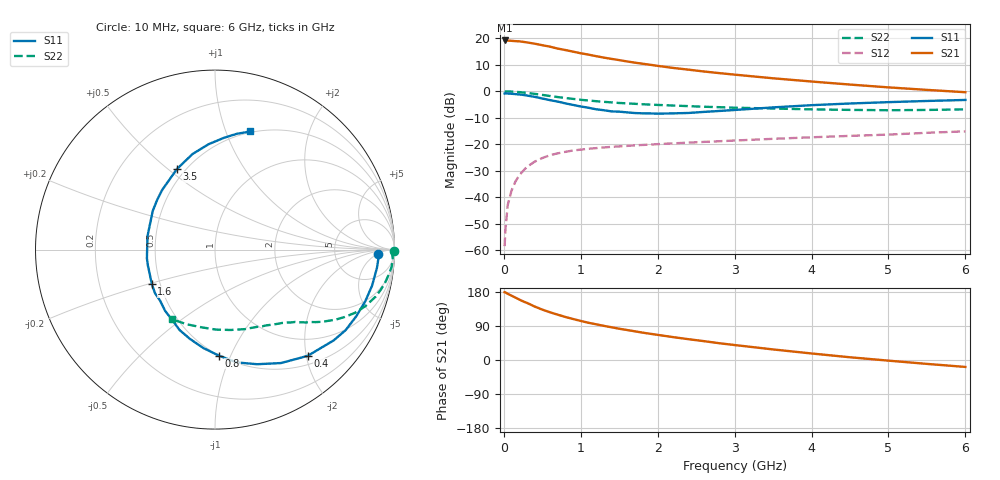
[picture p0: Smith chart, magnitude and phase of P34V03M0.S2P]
! SIEMENS Small Signal Semiconductors
! BFP181
! Si NPN RF Bipolar Junction Transistor in SOT143
! VCE = 4 V  IC = 3 mA
! Common Emitter S-Parameters:  March  1996
# GHz  S  MA  R  50
!  f  S11  S21  S12  S22
! GHz  MAG  ANG  MAG  ANG  MAG  ANG  MAG  ANG
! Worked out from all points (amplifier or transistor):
!   36 points, 10 MHz to 6 GHz, reference 50 ohm
!   highest |S21| = 19.2 dB at 10 MHz (marker M1)
!   |S21| within 3 dB of that: start of sweep to 690.9 MHz
!   unconditionally stable (mu >= 1): 2.142 GHz to end of sweep
!   at 250 MHz: K = 0.15, MSG = 24.3 dB, |S12| = -30.0 dB
!   at 1.4 GHz: K = 0.75, MSG = 16.6 dB, |S12| = -21.0 dB
!   at 6 GHz: K = 1.10, MAG = 5.5 dB, |S12| = -15.1 dB
!   lowest NFmin = 1.40 dB at 450 MHz
!   S11 on the Smith chart (normalised r, x): 10 MHz: 19, -5; 400 MHz: 0.66, -2.03; 800 MHz: 0.50, -0.91; 1.6 GHz: 0.45, -0.21; 3.5 GHz: 0.45, +0.54; 6 GHz: 0.49, +1.22
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0.01  0.9066 -1.5  9.092 178.9  0.0012 94.9  0.9953 -0.5
0.02  0.9122 -2.8  9.069 178.3  0.0024 86.2  0.987 -1.1
0.05  0.9081 -6.4  9.032 174.8  0.0071 89.4  0.9915 -2.9
0.1  0.898 -12.9  8.948 169.8  0.0134 82.4  0.9885 -5.7
0.2  0.87 -25.3  8.757 159.6  0.026 75.5  0.9653 -11.1
0.25  0.8554 -31.6  8.555 154.7  0.0315 72.0  0.9491 -13.8
0.4  0.7856 -48.9  7.902 141.2  0.047 63.0  0.8952 -20.6
0.5  0.7313 -59.8  7.398 133.0  0.0551 57.1  0.8558 -24.3
0.6  0.6804 -69.8  6.943 125.9  0.0623 53.2  0.815 -27.4
0.7  0.6399 -79.2  6.388 119.6  0.0676 49.5  0.779 -30.0
0.8  0.5913 -87.8  5.996 113.6  0.0721 45.9  0.7466 -32.1
1  0.517 -105.6  5.211 103.1  0.0794 41.0  0.6923 -35.7
1.1  0.4895 -113.8  4.92 98.2  0.0824 39.0  0.6694 -37.1
1.3  0.4398 -129.3  4.318 90.1  0.0873 35.7  0.6328 -39.8
1.6  0.4007 -151.5  3.658 79.2  0.0933 32.9  0.5924 -43.1
1.8  0.3843 -166.6  3.316 72.3  0.0972 31.8  0.5703 -45.4
2.2  0.3834 168.9  2.758 60.4  0.1043 29.1  0.5385 -50.3
2.8  0.4254 139.1  2.203 44.3  0.1143 26.6  0.5017 -58.5
3.5  0.4969 115.2  1.759 27.9  0.1269 23.8  0.4732 -69.5
4.5  0.5886 93.4  1.339 7.2  0.1442 19.3  0.4457 -89.4
5.5  0.6567 79.3  1.063 -10.3  0.1649 15.6  0.4449 -110.8
6  0.6867 73.4  0.96 -18.3  0.1756 12.7  0.4564 -121.9
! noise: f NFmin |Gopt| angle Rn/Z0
0.45  1.4  0.56  17  0.36
0.9  1.5  0.45  35  0.34
1.8  1.85  0.25  82  0.36
